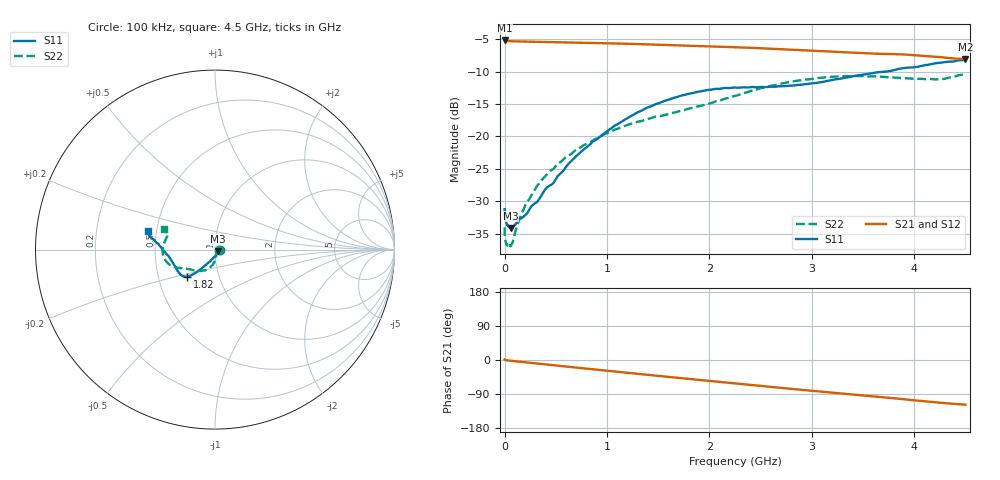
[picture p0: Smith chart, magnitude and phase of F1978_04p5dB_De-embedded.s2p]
! Integrated Device Technology
! Corporate Headquarters
! 6024 Silver Creek Valley Road
! San Jose, CA 95138  USA
! Phone:  1-408-284-8200
! Toll Free:  1-800-223-1366
! Webpage:  http://www.idt.com/
! Timing and RF Division
! 515 Groton Road, Suite 102
! Westford, MA 01886-6024
! Device:  F1978
! Description: 6-bit, 75 ohm, 0.5 dB Digital Step Attenuator
! Frequency:  5.0 MHz -  3.00 GHz
! Package:  4x4 mm QFN Plastic Package: 20 pin
! Ports:  2 RF, 11 DC
!  Pin  1  = D5 (16 dB)
!  Pin  2  = RF1  =  Port 1
!  Pin  3  = Serial Data In (DATA)
!  Pin  4  = Serial Clock (CLK)
!  Pin  5  = Serial Latch Enable (LE)
!  Pin  6  = VDD
!  Pin  7  = NC
!  Pin  8  = NC
!  Pin  9  = NC
!  Pin 10  = GND
!  Pin 11  = GND
!  Pin 12  = NC
!  Pin 13  = VMODE
!  Pin 14  = RF2  =  Port 2
!  Pin 15  = D4 (8 dB)
!  Pin 16  = D3 (4 dB)
!  Pin 17  = D2 (2 dB)
!  Pin 18  = NC
!  Pin 19  = D1 (1 dB)
!  Pin 20  = D0 (0.5 dB)
! State:  9
! Atten State:  4.5 dB
! Voltage:  +3.30 Volts
! Current:  0.566 mA
! Data:  The device was measured on a F1975 evaluation board which has
!  individual transmission lines to the RF pins.  Data was collected
!  using a calibrated network analyzer.  The evaluation board was
!  de-embedded using Automatic Fixture Removal (AFR).
!  The reference plane is the edge of the package pin.
! Misc:
!  Action Tracker AT0416
! Date Measured:  2018-02-08
! Date:  2018-03-26  MJV
! Note:
!  Integrated Device Technology supplies this data as a sample of measured
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# GHz S dB R 75
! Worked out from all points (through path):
!   291 points, 100 kHz to 4.5 GHz, reference 75 ohm
!   highest |S21| = -5.19 dB at 100 kHz (marker M1); lowest = -8.0 dB at 4.5 GHz (marker M2)
!   group delay of S21, straight-line fit = 73.8 ps
!   lowest |S11| = -34.1 dB at 60 MHz (marker M3), VSWR 1.04, Z = 77.7 - j1.39 ohm
!   |S11| at or under -10 dB: start of sweep to 3.726 GHz
!   |S22| runs from -36.9 to -10.3 dB; largest |S21 - S12| = 0.00021
!   S11 on the Smith chart (normalised r, x): 100 kHz: 1.06, -0.00; 1.82 GHz: 0.71, -0.22; 4.5 GHz: 0.45, +0.11
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0.0001  -31.24 -0.1  -5.19 1.2  -5.20 1.2  -34.03 0.2
0.0008  -32.21 -3.3  -5.23 1.0  -5.23 1.0  -35.01 -2.8
0.002  -32.52 -3.3  -5.24 0.8  -5.24 0.8  -35.47 -4.2
0.013  -33.16 -9.7  -5.27 -0.6  -5.27 -0.6  -36.44 -13.7
0.06  -34.12 -27.1  -5.31 -2.0  -5.31 -2.0  -36.90 -40.0
0.08  -33.93 -34.9  -5.32 -2.6  -5.32 -2.6  -36.30 -52.0
0.18  -32.45 -56.7  -5.37 -5.5  -5.36 -5.5  -31.42 -71.3
0.32  -30.08 -81.2  -5.41 -9.4  -5.41 -9.4  -27.58 -81.4
0.4  -28.12 -91.1  -5.43 -11.6  -5.43 -11.6  -26.09 -84.3
0.48  -27.13 -99.0  -5.45 -13.9  -5.45 -13.9  -24.96 -87.9
0.52  -26.10 -102.7  -5.46 -15.0  -5.46 -15.0  -24.26 -89.7
0.76  -22.18 -115.2  -5.53 -21.6  -5.53 -21.6  -21.51 -98.2
1.08  -18.30 -124.3  -5.65 -30.6  -5.65 -30.6  -18.94 -108.8
1.52  -14.79 -131.4  -5.86 -42.5  -5.86 -42.5  -16.86 -124.2
1.82  -13.37 -135.6  -6.03 -50.4  -6.02 -50.4  -15.64 -135.8
2.26  -12.47 -145.5  -6.25 -62.0  -6.24 -62.0  -13.70 -149.4
2.68  -12.26 -159.2  -6.52 -73.1  -6.52 -73.1  -11.92 -158.1
3.02  -11.80 -170.4  -6.78 -81.7  -6.78 -81.7  -11.08 -166.2
3.4  -10.73 180.0  -7.08 -91.1  -7.07 -91.1  -10.67 -177.3
3.76  -9.93 174.0  -7.29 -99.7  -7.28 -99.7  -10.88 173.1
4.22  -8.69 169.0  -7.70 -112.0  -7.70 -112.0  -11.21 161.7
4.5  -8.23 164.3  -8.04 -117.9  -8.04 -117.9  -10.30 157.6
